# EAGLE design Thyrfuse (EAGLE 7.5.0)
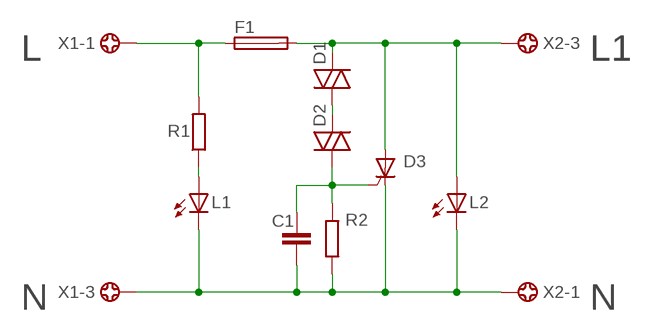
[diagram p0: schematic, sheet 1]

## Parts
C1  C-EU150-072X183  [C150-072X183]
D1  DIAC-DO35-10  [DO35-10]
D2  DIAC-DO35-10  [DO35-10]
D3  BTW68  [TOP3S-2]
F1  19559  [19559]
L1  LED5MM  [LED5MM]
L2  LED5MM  [LED5MM]
R1  R-EU_0617/22  [0617/22]
R2  R-EU_0309/12  [0309/12]
X1  5202-03-N-02  [5202-03-N-02]
X2  5202-03-N-02  [5202-03-N-02]

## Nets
N$1: D1.A D2.C
N$2: C1.1 D2.A D3.G R2.2
N$3: L1.A R1.1
N$4: F1.1 R1.2 X1.1
N$5: C1.2 D3.C L1.K(C) L2.K(C) R2.1 X1.3 X2.1
N$6: D1.C D3.A F1.2 L2.A X2.3
Unconnected: X1.2 X2.2

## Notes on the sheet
- L | L1
- N | N

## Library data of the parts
C1 = rcl:C-EU: CAPACITOR, European symbol
D1 D2 = diode:DIAC-: DIAC
D3 = triac:BTW68: THYRISTOR
F1 = fuse:19559: FUSE HOLDER; MPN: 55900000001; OC_FARNELL: 9516360; OC_NEWARK: 02P0286
L1 L2 = led:LED: LED
R1 R2 = rcl:R-EU_: RESISTOR, European symbol
X1 X2 = con-ebyelectro:5202-03-N-02: Barrier Blocks Sreies 5202 Source: http://www.ebyelectro.com/PDF/5202-XX-N-02.pdf; OC_FARNELL: unknown; OC_NEWARK: unknown

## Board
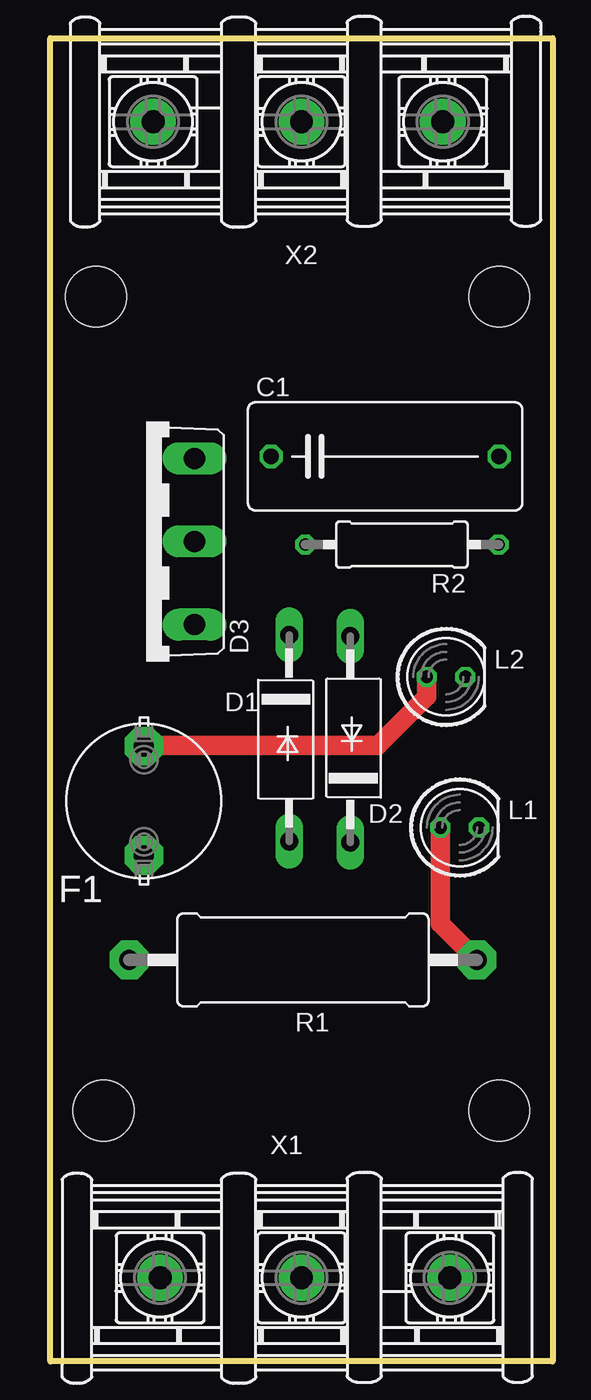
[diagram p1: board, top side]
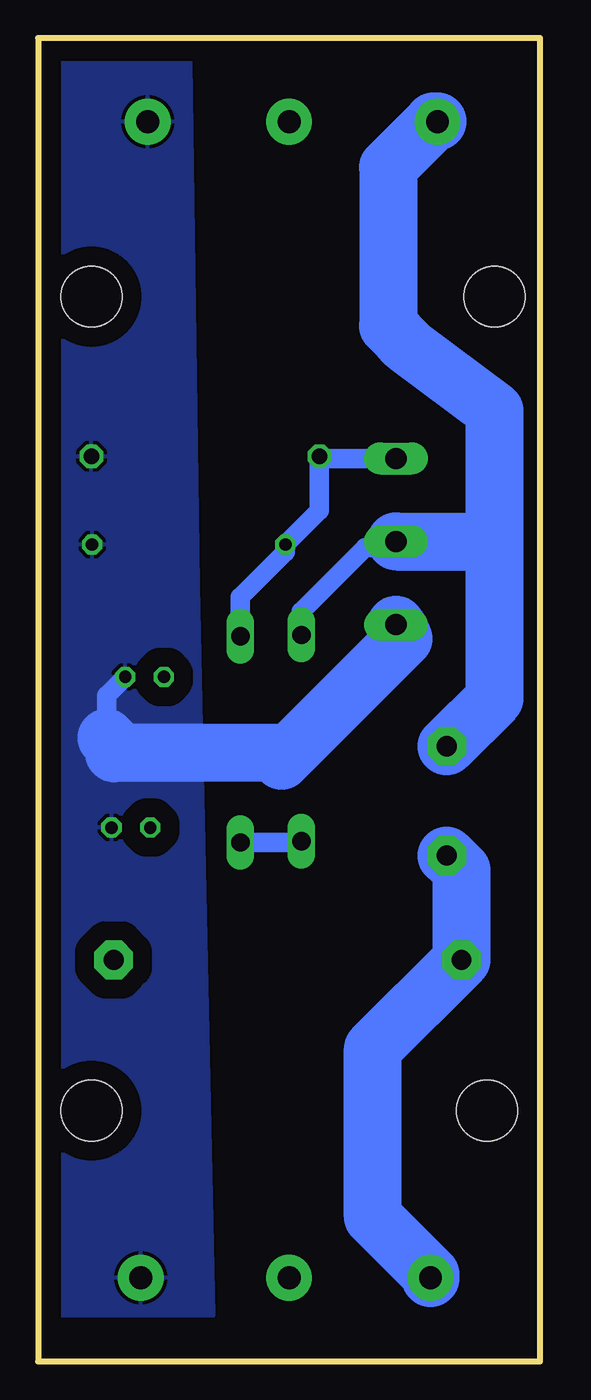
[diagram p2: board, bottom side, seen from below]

Size 33 x 87 mm. Coordinates in mm from the lower left corner, seen from the top.
Outline: 0,0 0,87 33,87 33,0 0,0
Copper layers (1*16): Top 0.035mm / dielectric 1.5mm / Bottom 0.035mm
Design rules "default": minimum track width 10mil, minimum drill 24mil, track to track 8mil, track to pad 8mil, pad to pad 8mil, via to via 8mil, smd to smd 8mil, copper to edge 40mil, drill to drill 8mil, minimum pad ring 10mil, minimum via ring 8mil, stop-mask expansion 4mil, vias tented up to drill 0mil, thermal gap 10mil
Holes 4 mm at 3.5,16.5 29.5,16.5 3,70 29.5,70

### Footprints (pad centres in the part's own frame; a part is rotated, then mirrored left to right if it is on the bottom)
C150-072X183 = drill 1.016 octagon: 1 -7.493,0; 2 7.493,0
DO35-10 = drill 1.2 long: A 8.18,0; C -5.38,0
TOP3S-2 = drill 1.397 long: A 0,-3.175; C -5.461,-3.175; G 5.461,-3.175
19559 = drill 1.321 pad 2.54 octagon: 1 -2.54,2.54; 2 2.54,-2.54
LED5MM = drill 0.813 octagon: A -1.27,0; K 1.27,0
0617/22 = drill 1.3 pad 2.54 octagon: 1 -11.43,0; 2 11.43,0
0309/12 = drill 0.813 octagon: 1 -6.35,0; 2 6.35,0
5202-03-N-02 = drill 1.5 pad 3: 1 -9.29,0; 2 0,0; 3 9.75,0

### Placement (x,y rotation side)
C1  22,59.5 0 top
D1  15.69,42.38 270 top
D2  19.7,39.5 90 top
D3  6.3,53.9 90 top
F1  6.15,36.85 135 top
L1  26.9,35.1 0 top
L2  26,45 0 top
R1  16.6,26.4 180 top
R2  23.1,53.7 180 top
X1  16.5,5.5 0 top
X2  16.5,81.5 180 top

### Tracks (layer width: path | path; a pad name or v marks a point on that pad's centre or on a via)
N$1
  Bottom 1.27: D2.C 15.77,34.12 D1.A
N$2
  Bottom 1.27: D2.A 19.7,50.25 16.75,53.2 R2.2 14.51,55.94 C1.1 14.37,59.36 D3.G
N$3
  Top 1.27: L1.A 25.63,28.8 R1.1
N$4
  Bottom 3.81: F1.1 5.17,32.28 R1.2 11,20.57 11,9.5 7.21,5.71 X1.1
N$5
  Bottom 1.27: 28.5,41 28.5,43.77 L2.K
  Bottom 3.81: 28.5,41 28,40.5 28,40 17,40 17,39.5 8.97,47.52 D3.C
  pour Bottom (isolate 1.27): 23,85.5 22.5,51 21.5,3 32.5,3 32.5,4.5 32,4.5 32,85.5
N$6
  Top 1.27: L2.A 24.73,43.73 21.5,40.5 6.2,40.5 F1.2
  Bottom 1.27: D1.C 15.69,49.31 11.5,53.5 9.88,53.5 D3.A
  Bottom 3.81: 3,53 3,43.59 F1.2 | 3,53 3,62.5 8.68,66.76 | 8.68,66.76 9,67 | X2.3 7,81.5 10,78.5 10,68.08 8.68,66.76 | D3.A 3.9,53.9 3,53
